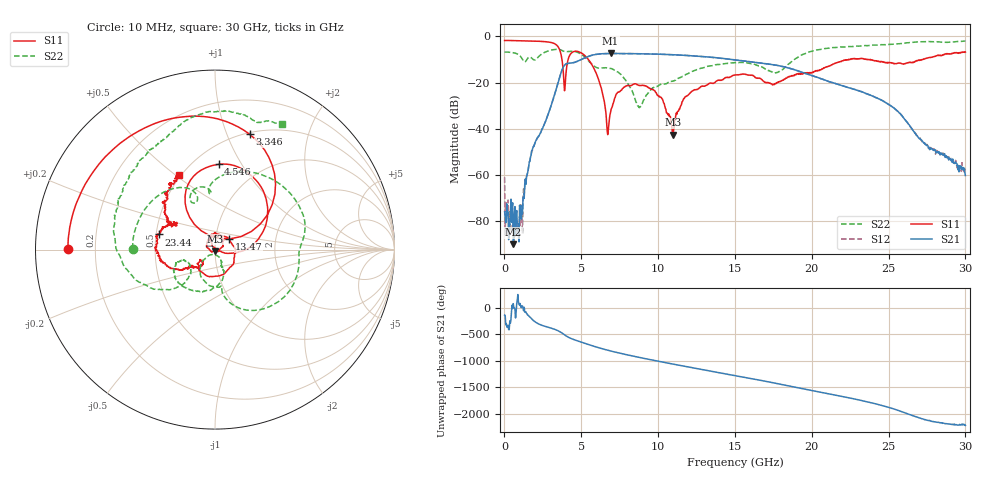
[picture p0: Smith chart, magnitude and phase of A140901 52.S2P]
!  2-Port S-parameters saved by WinCal
! VAR MeasName=S-Parameters (CALIBRATED_DATA) read from VNA (N5244A)
! VAR MeasDate=11/3/2014 9:35:58 AM
! VAR NAME=A140901 52
! VAR FILENAME=A140901 52.S2P
! VAR DATE=11/3/2014 9:35:58 AM
! VAR PHYS_PORTS=1,2
# Hz S RI R 50
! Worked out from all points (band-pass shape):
!   801 points, 10 MHz to 30 GHz, reference 50 ohm
!   highest |S21| = -7.33 dB at 6.908 GHz (marker M1); lowest = -89.9 dB at 572.3 MHz (marker M2)
!   |S21| within 3 dB of the highest: 4.881 GHz to 15.27 GHz (10.39 GHz wide, 103 % of centre)
!   lowest |S11| = -42.5 dB at 10.96 GHz (marker M3), VSWR 1.02, Z = 50 - j0.753 ohm
!   |S11| at or under -10 dB: 3.741 GHz to 4.143 GHz (401.6 MHz wide, 10.2 % of centre); 5.469 GHz to 22.38 GHz (16.91 GHz wide, 121 % of centre); 23.83 GHz to 27.23 GHz (3.4 GHz wide, 13.3 % of centre)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
!   |S22| runs from -30.8 to -2.0 dB; largest |S21 - S12| = 0.0025
!   S11 on the Smith chart (normalised r, x): 10 MHz: 0.10, +0.00; 3.346 GHz: 0.52, +1.21; 4.546 GHz: 0.65, +0.80; 13.47 GHz: 1.16, +0.14; 23.44 GHz: 0.52, +0.10; 30 GHz: 0.49, +0.52
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1e7  -0.8178 0.00284  -0.000107 -0.000121  0.000887 -0.000183  -0.4586 0.005
5.723125e8  -0.7957 0.1854  3.16e-06 3.17e-05  6.83e-05 -5.24e-05  -0.3626 0.2591
1.022162e9  -0.7432 0.3249  1.1e-05 0.000183  7.75e-05 8.18e-06  -0.158 0.3434
1.771912e9  -0.5918 0.5367  -0.00302 0.00143  -0.003 0.00144  -0.0372 0.3386
3.346388e9  0.1924 0.643  0.043 -0.0533  0.0432 -0.0536  0.4471 0.2774
3.9087e9  0.0244 0.0623  -0.2011 -0.1299  -0.2013 -0.1296  0.4738 0.00649
4.545988e9  0.0203 0.4751  -0.1362 0.2381  -0.136 0.2378  0.4175 -0.2268
5.033325e9  0.2553 0.3512  0.1033 0.3048  0.1029 0.3044  0.2216 -0.3387
5.895538e9  0.1826 0.00471  0.3999 -0.073  0.3992 -0.0719  0.0379 -0.2182
6.682775e9  0.00932 0.00179  0.1069 -0.4137  0.1073 -0.4129  -0.000537 -0.2077
6.9077e9  -0.0138 0.0185  -0.02 -0.4295  -0.0199 -0.4285  -0.0305 -0.2008
8.744588e9  0.0105 0.0869  -0.3541 0.2324  -0.3537 0.2318  -0.00757 -0.0283
1.001916e10  0.043 0.0281  0.1275 0.3948  0.1271 0.3942  0.0333 -0.0792
1.095635e10  -0.000204 -0.00754  0.3801 0.1332  0.3801 0.1335  0.0413 -0.0997
1.178108e10  -0.0476 0.0158  0.3493 -0.1722  0.3495 -0.1729  0.0483 -0.1415
1.346801e10  0.0786 0.0587  -0.1661 -0.3138  -0.1649 -0.3128  -0.0424 -0.2284
1.5005e10  0.038 -0.1409  -0.2916 0.1094  -0.2912 0.1094  -0.1751 -0.2078
1.762912e10  -0.0669 -0.067  0.2311 0.0681  0.2304 0.0682  -0.143 -0.0814
2.002832e10  -0.1395 -0.0905  -0.0772 -0.1191  -0.0765 -0.1201  -0.4557 -0.1527
2.343969e10  -0.3121 0.0846  0.0498 0.0337  0.05 0.0336  -0.4702 0.4242
2.501416e10  -0.2221 0.1492  0.00445 -0.0336  0.00467 -0.0337  -0.3085 0.5986
3e10  -0.1984 0.4153  0.00042 -0.000891  0.000598 -0.00125  0.374 0.7011
